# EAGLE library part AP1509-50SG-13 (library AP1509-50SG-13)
DiodesZetex, AP1509-50SG-13 DC-DC Converter 2A 8-Pin, SOP Source: Datasheet
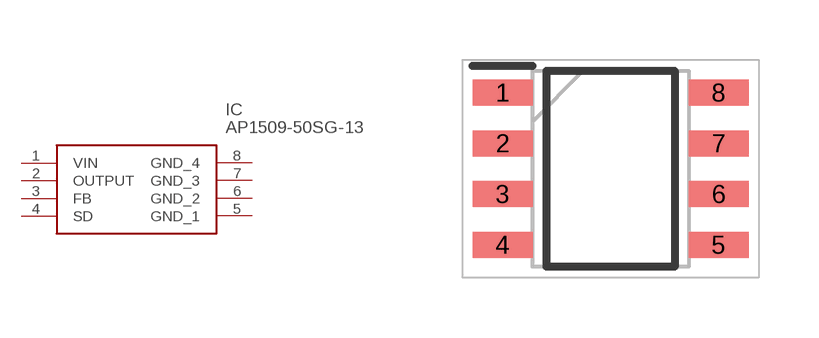
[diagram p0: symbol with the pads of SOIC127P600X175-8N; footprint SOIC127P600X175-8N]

Designator prefix IC

## AP1509-50SG-13 (Description: DiodesZetex, AP1509-50SG-13 DC-DC Converter 2A 8-Pin, SOP; Height: 1.75mm; Manufacturer_Name: Diodes Inc.; Manufacturer_Part_Number: AP1509-50SG-13; Mouser_Part_Number: 621-AP1509-50SG-13; Mouser_Price-Stock: https://www.mouser.co.uk/ProductDetail/Diodes-Incorporated/AP1509-50SG-13?qs=EJYhozv%252BYpwbI10CpTvwPw%3D%3D)  [SOIC127P600X175-8N]
1  VIN
2  OUTPUT
3  FB
4  SD
5  GND_1
6  GND_2
7  GND_3
8  GND_4

## Footprint SOIC127P600X175-8N (pad centres in mm)
SOP-8L
smd 1.5 x 0.65: 1 -2.7,1.905; 2 -2.7,0.635; 3 -2.7,-0.635; 4 -2.7,-1.905; 5 2.7,-1.905; 6 2.7,-0.635; 7 2.7,0.635; 8 2.7,1.905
